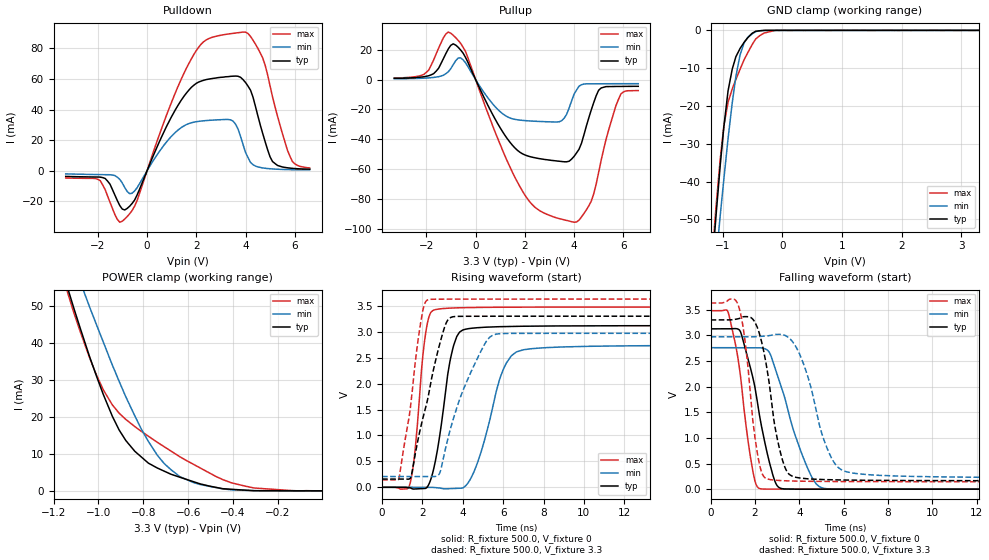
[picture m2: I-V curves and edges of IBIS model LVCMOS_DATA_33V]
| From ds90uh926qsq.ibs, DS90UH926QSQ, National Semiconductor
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[Model] LVCMOS_DATA_33V
Model_type 3-state
Enable Active-High
Vmeas = 1.65V
Cref = 0.0pF
Rref = 1.0e10
Vref = 0.0V
C_comp   2.75pF   2.32pF   3.18pF
[Voltage Range]   3.3V   2.97V   3.63V
[Temperature Range]   25.0   130.0   -40.0
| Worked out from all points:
|   slope of the pulldown table from 0 to 0.495 V, typ, clamps not added: 26.3 ohm
|   slope of the pullup table from 0 to 0.495 V, typ, clamps not added: 28.9 ohm
|   GND clamp passes 1 mA (typ) near -0.52 V on its own axis
|   POWER clamp passes 1 mA (typ) near -0.48 V on its own axis
|   rising waveform, R_fixture 500.0, V_fixture 0: 20-80 % time 700ps typ, 1.14ns min, 463ps max; typ from 0 V to 3.12 V
|   falling waveform, R_fixture 500.0, V_fixture 0: 20-80 % time 883ps typ, 1.21ns min, 633ps max; typ from 3.13 V to 0 V
|   rising waveform, R_fixture 500.0, V_fixture 3.3: 20-80 % time 1.08ns typ, 1.49ns min, 708ps max; typ from 0.159 V to 3.3 V
|   falling waveform, R_fixture 500.0, V_fixture 3.3: 20-80 % time 701ps typ, 1.07ns min, 518ps max; typ from 3.3 V to 0.162 V
[GND Clamp]
-3.3V     -551.2mA   -486.4mA   -619mA
-1.169V   -61.14mA   -71.51mA   -59.16mA
-1.109V   -48.96mA   -60.9mA    -46.58mA
-1.039V   -35.65mA   -48.93mA   -34.02mA
-978.3mV  -25.54mA   -39.39mA   -25.34mA
-907.9mV  -16.01mA   -28.64mA   -19.02mA
-837.6mV  -10.23mA   -19.13mA   -15.49mA
-706.9mV  -4.789mA   -6.49mA    -10.31mA
-636.5mV  -3.114mA   -3.224mA   -7.687mA
-445.6mV  -244.7uA   -327.8uA   -2.283mA
-103.9mV  2.352uA    -5.966uA   3.751uA
3.293V    1.162uA    0A         7.634uA
[POWER Clamp]
-3.3V     548.4mA    487.4mA    614mA
-1.139V   55.16mA    66.5mA     53.91mA
-1.109V   49.22mA    61.29mA    48mA
-1.079V   43.51mA    56.1mA     42.62mA
-1.039V   36.1mA     49.55mA    35.83mA
-978.3mV  26.05mA    40.2mA     27.29mA
-907.9mV  16.47mA    29.64mA    20.99mA
-777.3mV  7.485mA    13.36mA    14.75mA
-676.8mV  4.488mA    5.724mA    10.75mA
-576.2mV  2.468mA    2.234mA    7.162mA
-405.4mV  408.8uA    263.5uA    2.141mA
-3.35mV   -590.9nA   -7.985uA   -29.37uA
[Pullup]
-3.3V     799.7uA    508.2uA    1.021mA
-2.003V   2.146mA    986.4uA    4.681mA
-1.008V   22.85mA    7.191mA    30.99mA
-606.4mV  19.72mA    14.48mA    24.18mA
891.2mV   -29.36mA   -19.87mA   -39.15mA
1.997V    -50.43mA   -27.47mA   -77.24mA
3.494V    -54.86mA   -27.54mA   -93.44mA
3.997V    -51.42mA   -9.751mA   -95.45mA
4.69V     -20.51mA   -2.871mA   -81.52mA
4.992V    -7.209mA   -2.848mA   -62.19mA
5.896V    -4.639mA   -2.808mA   -9.618mA
6.6V      -4.554mA   -2.795mA   -7.412mA
[Pulldown]
-3.3V     -3.683mA   -2.031mA   -4.727mA
-1.903V   -4.132mA   -2.497mA   -6.372mA
-1.008V   -24.97mA   -7.892mA   -33.01mA
-606.4mV  -21.35mA   -14.67mA   -25.96mA
891.2mV   32.17mA    20.78mA    40.6mA
1.997V    57.12mA    32.07mA    78.54mA
3.394V    61.73mA    33.29mA    89.61mA
3.896V    59.57mA    17.05mA    90.64mA
4.69V     24.51mA    1.879mA    73.84mA
5.092V    6.034mA    1.201mA    48.23mA
5.896V    1.588mA    707.4uA    6.09mA
6.6V      1.067mA    678.5uA    1.859mA
[Rising Waveform]
R_fixture=500.0
V_fixture=0
V_fixture_min=0
V_fixture_max=0
0s        24.71nV    508.9nV    67.81nV
1.35ns    -8.956mV   486.1nV    26.26mV
2.2ns     -11.95mV   2.02uV     3.068V
2.75ns    732.9mV    -9.191mV   3.435V
3.35ns    2.399V     -26.18mV   3.455V
3.8ns     2.969V     -20mV      3.462V
4.75ns    3.078V     495mV      3.469V
6.05ns    3.099V     2.308V     3.473V
7ns       3.106V     2.652V     3.474V
49.98ns   3.12V      2.746V     3.477V
[Falling Waveform]
R_fixture=500.0
V_fixture=0
V_fixture_min=0
V_fixture_max=0
0s        3.126V     2.759V     3.48V
800ps     3.126V     2.759V     3.44V
1.35ns    3.068V     2.759V     2.195V
1.85ns    2.274V     2.759V     486.3mV
2.25ns    1.327V     2.757V     7.791mV
2.65ns    525.1mV    2.666V     956.7uV
3.05ns    44.06mV    2.169V     626.8uV
4.35ns    635.6uV    433mV      290uV
5.2ns     400.8uV    10.27mV    198.4uV
49.98ns   5.596uV    14.57uV    1.497uV
[Rising Waveform]
R_fixture=500.0
V_fixture=3.3
V_fixture_min=2.97
V_fixture_max=3.63
0s        159mV      207.3mV    143.3mV
850ps     159mV      207.3mV    188.9mV
1.45ns    221.6mV    207.3mV    1.689V
2ns       1.299V     207.3mV    3.369V
2.35ns    1.88V      207.3mV    3.623V
2.85ns    2.754V     267mV      3.628V
3.3ns     3.245V     998.4mV    3.629V
4.6ns     3.299V     2.387V     3.629V
5.7ns     3.299V     2.956V     3.63V
49.98ns   3.3V       2.97V      3.63V
[Falling Waveform]
R_fixture=500.0
V_fixture=3.3
V_fixture_min=2.97
V_fixture_max=3.63
0s        3.3V       2.97V      3.63V
1.25ns    3.323V     2.97V      3.584V
1.55ns    3.365V     2.97V      2.896V
2.15ns    3.102V     2.976V     600.4mV
2.7ns     1.868V     2.999V     185.7mV
3.1ns     797.4mV    3.019V     168.6mV
3.55ns    286.2mV    2.944V     160.4mV
5.35ns    184mV      698.1mV    150mV
6.4ns     175.5mV    314.3mV    148mV
49.98ns   162mV      216.6mV    144.5mV
[Ramp]
R_load = 500.0
dV/dt_r   1.872022E0/7E-10   1.647461E0/1.15E-9   2.086495E0/4.5E-10
dV/dt_f   1.88279E0/7E-10   1.652063E0/1.05E-9   2.091306E0/5.5E-10
